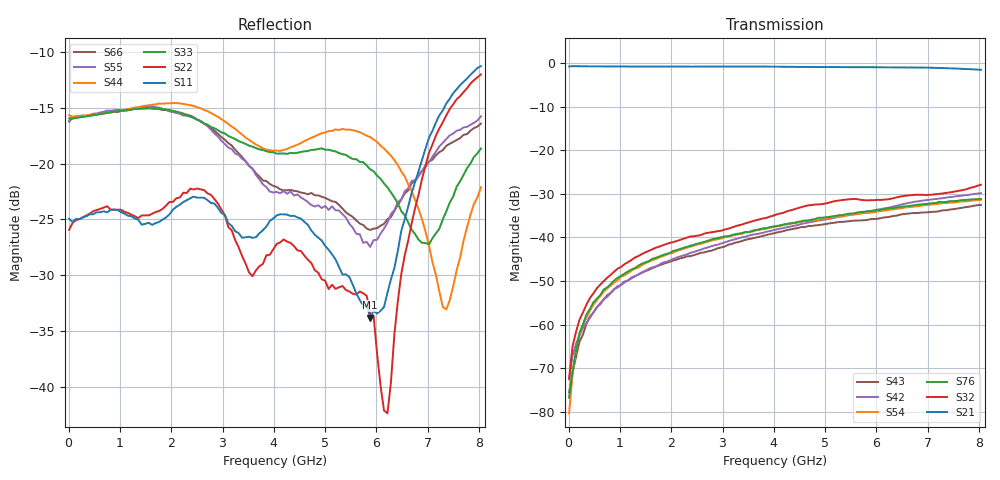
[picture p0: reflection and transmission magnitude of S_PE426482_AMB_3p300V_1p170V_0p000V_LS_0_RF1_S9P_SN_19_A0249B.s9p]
! Device ID: PE426482
! File Path: z:\PE426482\Final Char Data\room\AMB\3p300\LS_0_RF1\PE426482_AMB_3p300V_1p170V_0p000V_LS_0_RF1_S9P_SN_19_A0249B.s9p
! Serial: 19
! Lot: A0249B
! Temp: AMB
! VDD: 3.300
! VSS: 0.000
! Control_Hi: 1.170
! Control_Lo: 0.000
! Logic State: LS_0_RF1
! Port 1:
! Port 2:
! Port 3:
! Port 4:
! Port 5:
! Port 6:
! Port 7:
! Port 8:
! Port 9:
! ThroughPath:1-2
! IDD: 0.0001062657
! ISS/IDD2: 9.5e-009
! IDMM3/IDD3: -2.535e-007
! Comment:
#  Hz  S  RI  R  50
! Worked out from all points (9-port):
!   120 points, 10 MHz to 8.037 GHz, reference 50 ohm
!   strongest paths, dB at 10 MHz, 2.034 GHz, 4.057 GHz, 6.08 GHz, 8.037 GHz:
!     S21: -0.8, -0.8, -0.8, -1.0, -1.6
!     S32: -72.3, -41.1, -34.7, -31.4, -27.9
!     S76: -76.8, -43.1, -37.4, -33.7, -31.2
!     S54: -80.3, -43.5, -37.5, -33.9, -31.4
!     S42: -72.6, -45.0, -38.2, -33.5, -29.9
!     S43: -75.5, -45.3, -38.9, -35.6, -32.5
!   lowest |S11| = -33.8 dB at 5.878 GHz (marker M1), VSWR 1.04, Z = 48.8 - j1.63 ohm
!   |S11| at or under -10 dB: start of sweep to end of sweep
